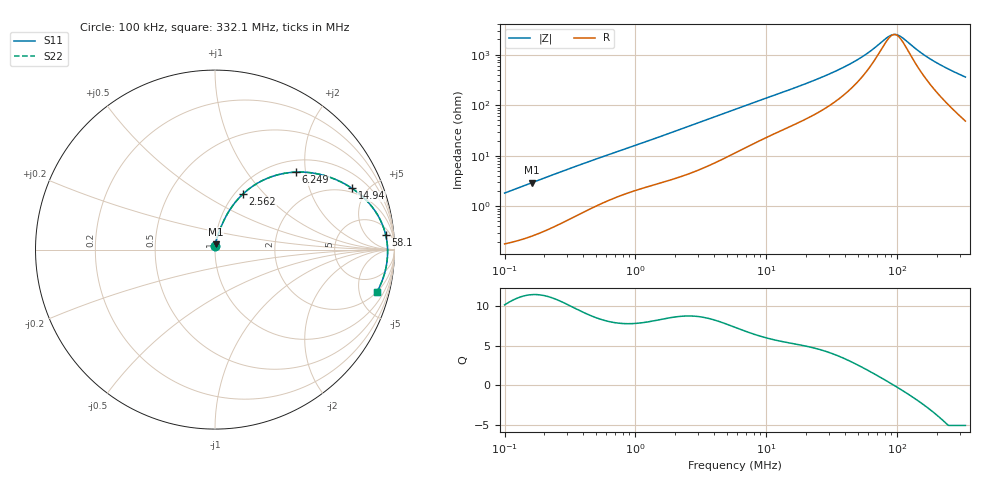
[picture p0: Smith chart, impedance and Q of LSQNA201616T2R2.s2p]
! LSQNA201616T2R2  S-PARAMETER MODEL  ( General Type )
! Model Generated by TAIYO YUDEN Corporation (http://www.ty-top.com)
! Version 2.0
! TAIYO YUDEN Control No. 100810NF25SB-FKC
! Copyright(c) 2007 TAIYO YUDEN CO.,LTD. All Rights Reserved.
! Product Description (link to TY-COMPAS)
! https://ds.yuden.co.jp/TYCOMPAS/or/detail?pn=LSQNA201616T2R2M&u=M
! Products Name : Inductors
! Characteristics :
!  Inductance : 2.2 uH , SRF(min) : 70 MHz , DC Resistance(max) : 0.169 Ohm
!  Rated Current : Saturation :510 mA , Temp Rise : 1000 mA (40 degC)
!  Case Size : 2.0 x 1.6 / 0.079 x 0.063 [mm/inch] , Thickness : 1.6 / 0.063 [mm/inch]
!  (Conditions: Temperature = 25 degC , DC Bias Current/Voltage = 0A / 0V)
! External Node Assignments :
!  1  o---GGG---o  2
! GND o---------o GND
! Frequency Range : 0.1MHz  -  332.076389MHz  [ 402 STEP ]
# MHz S RI R 50
! Freq[MHz].  S11 Real  S11 Imag  S21 Real  S21 Imag  S12 Real  S12 Imag  S22 Real  S22 Imag
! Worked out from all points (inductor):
!   401 points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, 100 kHz to 332.1 MHz, reference 50 ohm
!   read as one part in series: L = 2.88 uH near 104.1 kHz
!   highest Q = 11.4 at 162.7 kHz (marker M1), where L = 2.87 uH
!   self-resonance near 95.07 MHz
!   S11 on the Smith chart (normalised r, x): 100 kHz: 1.00, +0.04; 2.562 MHz: 1.09, +0.76; 6.249 MHz: 1.25, +1.78; 14.94 MHz: 1.74, +3.95; 58.1 MHz: 10, +18; 332.1 MHz: 1.97, -7.14
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0.1  0.00212 0.0181  0.9979 -0.0181  0.9979 -0.0181  0.00212 0.0181
0.162658  0.00343 0.0292  0.9966 -0.0292  0.9966 -0.0292  0.00343 0.0292
0.388873  0.0118 0.0665  0.9882 -0.0665  0.9882 -0.0665  0.0118 0.0665
0.806712  0.0329 0.1251  0.9671 -0.1251  0.9671 -0.1251  0.0329 0.1251
1.512219  0.075 0.2094  0.925 -0.2094  0.925 -0.2094  0.075 0.2094
2.561505  0.1554 0.3094  0.8446 -0.3094  0.8446 -0.3094  0.1554 0.3094
3.764905  0.2603 0.3828  0.7397 -0.3828  0.7397 -0.3828  0.2603 0.3828
5.762607  0.4195 0.4296  0.5805 -0.4296  0.5805 -0.4296  0.4195 0.4296
6.2493  0.4524 0.4319  0.5476 -0.4319  0.5476 -0.4319  0.4524 0.4319
9.185233  0.6048 0.414  0.3952 -0.414  0.3952 -0.414  0.6048 0.414
14.94048  0.7628 0.3418  0.2372 -0.3418  0.2372 -0.3418  0.7628 0.3418
22.4092  0.8555 0.2618  0.1445 -0.2618  0.1445 -0.2618  0.8555 0.2618
38.73557  0.9274 0.1519  0.0726 -0.1519  0.0726 -0.1519  0.9274 0.1519
48.41099  0.943 0.1109  0.057 -0.1109  0.057 -0.1109  0.943 0.1109
58.09942  0.9517 0.0794  0.0483 -0.0794  0.0483 -0.0794  0.9517 0.0794
87.14324  0.9611 0.0137  0.0389 -0.0137  0.0389 -0.0137  0.9611 0.0137
96.43822  0.9617 -0.00227  0.0383 0.00227  0.0383 0.00227  0.9617 -0.00227
104.5831  0.9618 -0.0151  0.0382 0.0151  0.0382 0.0151  0.9618 -0.0151
147.6095  0.9576 -0.0717  0.0424 0.0717  0.0424 0.0717  0.9576 -0.0717
180.7778  0.9511 -0.1079  0.0489 0.1079  0.0489 0.1079  0.9511 -0.1079
245.0144  0.9332 -0.1687  0.0668 0.1687  0.0668 0.1687  0.9332 -0.1687
332.0764  0.9007 -0.2387  0.0993 0.2387  0.0993 0.2387  0.9007 -0.2387
